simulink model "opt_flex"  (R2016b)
settings: Solver=ode4  StartTime=0.0  StopTime=trun2  FixedStep=step_sz  RelTol=1e-7  EnableMultiTasking=on
PreLoadFcn:
  | env_timeOpt2nd
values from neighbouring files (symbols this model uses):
  A = [0 1;-(w)^2 0;]    [figure_4.m]    (also in figure_3.m; figure_2.m; results.m)
  alpha = .5    (= 0.5)    [figure_4.m]    (also in figure_3.m = 0.8; figure_2.m; results.m = 0.7)
  B = [0; bo]    [figure_4.m]    (also in figure_3.m; figure_2.m; results.m)
  bo = 1.8276*10^7    (= 18276000)    [figure_4.m]    (also in figure_3.m; figure_2.m; results.m)
  c = bo/w^2    (= 4.59233914625)    [figure_4.m]    (also in figure_3.m; figure_2.m; results.m)
  k1 = (c-xl)/(c*xl)    (= 1.95978557188)    [figure_4.m]    (also in figure_3.m = 0.508092555672; figure_2.m; results.m = 0.819169630574; switching_curves_comp_func.m = (c-xl)/(c*xl))
  k2 = sqrt(2*c*alpha*xl-alpha*xl^2)/(alpha*w*c*xl)    [figure_4.m]    (also in figure_3.m; figure_2.m; results.m; switching_curves_comp_func.m)
  T = 1    [figure_4.m]    (also in figure_3.m; figure_2.m; results.m; switching_curves_comp_func.m)
  w = 2*pi*3.175*10^2    (= 1994.91133503)    [figure_4.m]    (also in figure_3.m; figure_2.m; results.m; plotshaded.m = varargout)
  x1Tol = .001*c    (= 0.00459233914625)    [figure_4.m]    (also in figure_2.m = 2.6e-12; results.m)
  x2_bound = 10*bo/w    (= 91613.0941716)    [figure_4.m]    (also in figure_3.m; figure_2.m = 18322.6188343; results.m = 18322.6188343)
  xl = .1*c    (= 0.459233914625)    [figure_4.m]    (also in figure_3.m = 1.37770174388; figure_2.m; results.m = 0.964391220713)
  Xo = [8.665 4229]    [figure_4.m]    (also in figure_3.m = [2*c, 0]; figure_2.m = [curves_optx1(k), curves_optx2(k)]; results.m = [3.0*c,0])
libraries: simulink x2

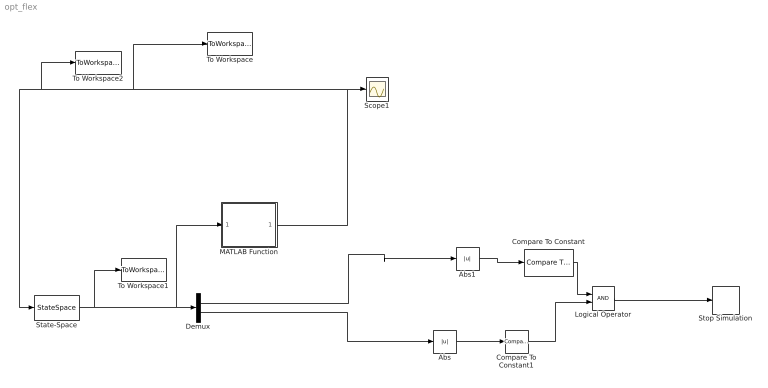
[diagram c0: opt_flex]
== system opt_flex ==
  Abs : Abs
  Abs1 : Abs
  Compare To Constant : simulink/Logic and Bit Operations/Compare To Constant  relop=<  const=x1Tol  OutDataTypeStr=boolean
  Compare To Constant1 : simulink/Logic and Bit Operations/Compare To Constant  relop=<=  const=.1  OutDataTypeStr=boolean
  Demux : Demux  Outputs=[1, 1]
  Logical Operator : Logic  AllPortsSameDT=off  OutDataTypeStr=boolean
  MATLAB Function : MATLAB Function  TreatAsAtomicUnit=on
  Scope1 : Scope
  State-Space : StateSpace  A=A  B=B  C=eye(2)  D=[0;0]  X0=Xo  ContinuousStateAttributes="{'xx1',  'xx2'}"
  Stop Simulation : Stop
  To Workspace : ToWorkspace  VariableName=control_flex_opt  SampleTime=-1
  To Workspace1 : ToWorkspace  VariableName=stateX  SaveFormat=Timeseries  SampleTime=-1
  To Workspace2 : ToWorkspace  VariableName=u_t  SaveFormat=Timeseries  SampleTime=-1
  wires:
  Demux/1 -> Abs1/1
  Demux/2 -> Abs/1
  State-Space/1 -> To Workspace1/1, MATLAB Function/1(u), Demux/1
  MATLAB Function/1(y) -> Scope1/1, To Workspace/1, To Workspace2/1, State-Space/1
  Compare To Constant/1 -> Logical Operator/1
  Logical Operator/1 -> Stop Simulation/1
  Compare To Constant1/1 -> Logical Operator/2
  Abs/1 -> Compare To Constant1/1
  Abs1/1 -> Compare To Constant/1

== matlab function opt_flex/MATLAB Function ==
function y = fcn(u, bo, w, c, xl, k1, k2, T, alpha, x2_bound)
%#codegen



fArg=u(1)/c;
fpart=fArg-fix(fArg);

%% compute x1_bar
if (mod(sign(u(1)/c)*floor(abs(u(1)/c)), 2)==0);
        x1_bar=c-abs(fpart*c);
    else
        x1_bar=fpart*c;
end

%% compute control
% <x2_bound
% if( abs(u(1)) < 2*c & abs(u(1)) > xl )
%       Fptos= sign(u(1)) *( w*sqrt(alpha*2*c*abs(u(1)) -alpha*u(1)^2) -1/k2);
%       control=sat( k2*(-Fptos -u(2)), T);
%  elseif(abs(u(1)) <xl )
%      Fptos=(k1/k2)*u(1);
%      control=sat( k2*(-Fptos -u(2)), T);
% 
% elseif( sign(u(1)*u(2))==1 | (u(2)/w)^2 <= (c^2 - x1_bar^2) )
%     control=-sign(u(1));
% else
%     control=sign(u(1));
% end
fto = sign(u(1))*w*sqrt(c^2 - x1_bar^2);
control = -sign(u(2) + fto);

y=[control];
